| IBIS file qfp100_1p8v.ibs generated by Viper version: 2020.12.17
[IBIS Ver]   5.0
[Comment Char]   |_char
[File Name]   qfp100_1p8v.ibs
[File Rev]   1.3
[Date]   Thu Dec 17 17:51:14 2020
[Source]   NXP Viper 2020.12.17
[Notes]
[Disclaimer] IMPORTANT NOTICE
  This information is provided on an AS IS basis and without warranty.
  IN NO EVENT SHALL NXP BE LIABLE FOR INCIDENTAL OR CONSEQUENTIAL
  DAMAGES ARISING FROM USE OF THIS INFORMATION. THIS DISCLAIMER OF
  WARRANTY EXTENDS TO THE USER OF THE INFORMATION, AND TO THEIR CUSTOMERS
  OR USERS OF PRODUCTS  AND IS IN LIEU OF ALL WARRANTIES WHETHER EXPRESS,
  IMPLIED, OR STATUTORY, INCLUDING IMPLIED WARRANTIES OF MERCHANTABILITY
  OR FITNESS FOR PARTICULAR PURPOSE.
  NXP does not represent or warrant that the information furnished
  hereunder is free of infringement of any third party patents,
  copyrights, trade secrets, or other intellectual property rights.
  NXP does not represent or warrant that the information is free of
  defect, or that it meets any particular standard, requirements or need
  of the user of the infomation or their customers.
  NXP reserves the right to change the information in this file
  without notice.
   http://www.nxp.com
[Copyright]   (C) Copyright NXP 2004 - 2020, All Rights Reserved.
|   qfp100
[Component]   qfp100
[Manufacturer]   NXP
[Package]
| variable   typ   min   max
R_pkg   0.20929   0.13326   0.23511
L_pkg   4.766e-09   4.182e-09   5.347e-09
C_pkg   4.363e-13   3.854e-13   5.112e-13
[Pin] signal_name   model_name   R_pin   L_pin   C_pin
1   P2_1   gpio   0.22359   5.036e-09 4.838e-13
2   OPAMP2_INN   NC   0.21497   4.843e-09 4.817e-13
3   P1_24   gpio   0.21478   4.857e-09 4.678e-13
4   P1_7   gpio   0.218   4.970e-09 4.597e-13
5   P0_1   gpio   0.2137   4.924e-09 4.401e-13
6   P1_0   gpio   0.21171   4.894e-09 4.292e-13
7   ADC1IN1B   NC   0.20848   4.761e-09 4.267e-13
8   ADC1IN1A   NC   0.19449   4.500e-09 4.295e-13
9   P0_11   gpio   0.19424   4.487e-09 4.205e-13
10   P0_12   gpio   0.19613   4.592e-09 4.148e-13
11   P1_20   gpio   0.20355   4.669e-09 3.944e-13
12   VDDE_0   POWER   NA   NA   NA
13   VDDA   POWER   NA   NA   NA
14   VREF_OUT   NC   NA   NA   NA
15   VREFP   NC   NA   NA   NA
16   VREFN   NC   NA   NA   NA
17   VSSA   GND   NA   NA   NA
18   VSSA   GND   NA   NA   NA
19   P0_23   gpio   0.20931   4.770e-09 4.124e-13
20   P0_16   gpio   0.21094   4.801e-09 4.247e-13
21   P0_10   gpio   0.21059   4.789e-09 4.343e-13
22   P0_15   gpio   0.20486   4.653e-09 4.661e-13
23   P0_31   gpio   0.21132   4.793e-09 4.798e-13
24   P2_0   gpio   0.22019   4.963e-09 4.885e-13
25   P1_9   gpio   0.22303   5.076e-09 4.722e-13
26   P0_8   gpio   0.22345   5.084e-09 4.854e-13
27   OPAMP0_INN   NC   0.21484   4.864e-09 4.951e-13
28   P0_27   gpio   0.20723   4.771e-09 4.735e-13
29   OPAMP1_INN   NC   0.21128   4.865e-09 4.521e-13
30   P1_19   gpio   0.20854   4.878e-09 4.401e-13
31   DAC0_OUT   NC   0.206   4.816e-09 4.186e-13
32   XTAL32M_N   NC   0.20742   4.770e-09 4.123e-13
33   XTAL32M_P   NC   0.19377   4.497e-09 4.206e-13
34   RESETN   gpio   0.19458   4.551e-09 4.119e-13
35   P1_5   gpio   0.19484   4.525e-09 4.071e-13
36   P1_8   gpio   0.2033   4.733e-09 3.981e-13
37   P1_21   gpio   0.20532   4.769e-09 3.889e-13
38   VDD_CORE   POWER   NA   NA   NA
39   P1_10   gpio   0.20393   4.722e-09 3.877e-13
40   P1_22   gpio   0.20253   4.623e-09 3.978e-13
41   P0_17   gpio   0.1965   4.443e-09 4.056e-13
42   P0_7   gpio   0.19935   4.370e-09 4.202e-13
43   VDDE_2   POWER   NA   NA   NA
44   VSS_MAIN_PWR   GND   NA   NA   NA
45   VSS_MAIN   GND   NA   NA   NA
46   LX   NC   0.13326   4.182e-09 5.112e-13
47   VDD_MAIN_PWR   NC   NA   NA   NA
48   VDD_MAIN   NC   NA   NA   NA
49   P1_23   gpio   0.22732   4.889e-09 4.839e-13
50   P1_6   gpio   0.23364   5.213e-09 4.781e-13
51   XTAL32K_P   NC   0.22796   4.990e-09 4.836e-13
52   XTAL32K_N   NC   0.2234   4.815e-09 4.954e-13
53   VBAT   NC   NA   NA   NA
54   P0_0   gpio   0.22115   4.940e-09 4.485e-13
55   P0_9   gpio   0.21453   4.836e-09 4.446e-13
56   P0_18   gpio   0.21091   4.806e-09 4.328e-13
57   P1_14   gpio   0.20872   4.790e-09 4.186e-13
58   P1_13   gpio   0.19633   4.586e-09 4.144e-13
59   P1_1   gpio   0.1964   4.593e-09 4.130e-13
60   P0_26   gpio   0.19597   4.536e-09 4.137e-13
61   P1_2   gpio   0.20506   4.751e-09 4.044e-13
62   P1_3   gpio   0.2073   4.774e-09 3.901e-13
63   VDDE_4   POWER   NA   NA   NA
64   P1_18   gpio   0.20968   4.757e-09 3.946e-13
65   P1_30   gpio   0.20872   4.724e-09 4.090e-13
66   P0_28   gpio   0.20197   4.577e-09 4.097e-13
67   P1_12   gpio   0.20002   4.567e-09 4.142e-13
68   P1_26   gpio   0.20357   4.672e-09 4.224e-13
69   P0_24   gpio   0.21269   4.876e-09 4.152e-13
70   P0_13   iic   0.21536   4.889e-09 4.354e-13
71   P0_14   iic   0.2194   4.920e-09 4.378e-13
72   P1_28   gpio   0.22057   4.931e-09 4.474e-13
73   P0_20   gpio   0.2194   4.845e-09 4.688e-13
74   VDDE_4   POWER   NA   NA   NA
75   P1_4   gpio   0.23319   5.014e-09 4.840e-13
76   P0_21   gpio   0.23511   5.347e-09 4.796e-13
77   P1_25   gpio   0.22334   4.949e-09 4.943e-13
78   P0_22   gpio   0.21505   4.857e-09 4.731e-13
79   P0_25   gpio   0.22039   4.977e-09 4.534e-13
80   P1_29   gpio   0.21599   4.949e-09 4.368e-13
81   P0_2   gpio   0.21746   4.944e-09 4.295e-13
82   P1_15   gpio   0.21349   4.812e-09 4.315e-13
83   P0_19   gpio   0.19872   4.518e-09 4.316e-13
84   P0_3   gpio   0.20028   4.498e-09 4.141e-13
85   VDDE_4   POWER   NA   NA   NA
86   P1_27   gpio   0.20706   4.743e-09 3.880e-13
87   P0_4   gpio   0.2043   4.699e-09 3.854e-13
88   P1_16   gpio   0.19807   4.528e-09 4.115e-13
89   P0_6   gpio   0.20532   4.850e-09 3.921e-13
90   P0_5   gpio   0.20447   4.757e-09 3.984e-13
91   P1_17   gpio   0.19816   4.603e-09 4.099e-13
92   P1_31   gpio   0.19768   4.570e-09 4.240e-13
93   P0_29   gpio   0.20649   4.690e-09 4.278e-13
94   P1_11   gpio   0.21516   4.752e-09 4.253e-13
95   P0_30   gpio   0.21957   4.695e-09 4.329e-13
96   VDDE_4   POWER   NA   NA   NA
97   VDD3V3_USB_FS   POWER   NA   NA   NA
98   USB_FS_DP_DM_IOP   NC   0.21894   4.661e-09 4.667e-13
99   USB_FS_DP_DM_IOM   NC   0.22487   4.721e-09 4.843e-13
100   VSS_USB_FS   GND   NA   NA   NA
101   VSS   GND   NA   NA   NA
[Pin Mapping]   pulldown_ref   pullup_ref
1   VSS   VDDE_0
2   NC   NC
3   VSS   VDDE_0
4   VSS   VDDE_0
5   VSS   VDDE_0
6   VSS   VDDE_0
7   NC   NC
8   NC   NC
9   VSS   VDDE_0
10   VSS   VDDE_0
11   VSS   VDDE_0
12   NC   VDDE_0
13   NC   VDDA
14   NC   NC
15   NC   NC
16   NC   NC
17   VSSA   NC
18   VSSA   NC
19   VSS   VDDE_0
20   VSS   VDDE_0
21   VSS   VDDE_0
22   VSS   VDDE_0
23   VSS   VDDE_0
24   VSS   VDDE_0
25   VSS   VDDE_0
26   VSS   VDDE_0
27   NC   NC
28   VSS   VDDE_0
29   NC   NC
30   VSS   VDDE_0
31   NC   NC
32   NC   NC
33   NC   NC
34   VSS   VDDE_2
35   VSS   VDDE_2
36   VSS   VDDE_2
37   VSS   VDDE_2
38   NC   VDD_CORE
39   VSS   VDDE_2
40   VSS   VDDE_2
41   VSS   VDDE_2
42   VSS   VDDE_2
43   NC   VDDE_2
44   VSS_MAIN_PWR   NC
45   VSS_MAIN   NC
46   NC   NC
47   NC   NC
48   NC   NC
49   VSS   VDDE_2
50   VSS   VDDE_2
51   NC   NC
52   NC   NC
53   NC   NC
54   VSS   VDDE_4
55   VSS   VDDE_4
56   VSS   VDDE_4
57   VSS   VDDE_4
58   VSS   VDDE_4
59   VSS   VDDE_4
60   VSS   VDDE_4
61   VSS   VDDE_4
62   VSS   VDDE_4
63   NC   VDDE_4
64   VSS   VDDE_4
65   VSS   VDDE_4
66   VSS   VDDE_4
67   VSS   VDDE_4
68   VSS   VDDE_4
69   VSS   VDDE_4
70   VSS   VDDE_4
71   VSS   VDDE_4
72   VSS   VDDE_4
73   VSS   VDDE_4
74   NC   VDDE_4
75   VSS   VDDE_4
76   VSS   VDDE_4
77   VSS   VDDE_4
78   VSS   VDDE_4
79   VSS   VDDE_4
80   VSS   VDDE_4
81   VSS   VDDE_4
82   VSS   VDDE_4
83   VSS   VDDE_4
84   VSS   VDDE_4
85   NC   VDDE_4
86   VSS   VDDE_4
87   VSS   VDDE_4
88   VSS   VDDE_4
89   VSS   VDDE_4
90   VSS   VDDE_4
91   VSS   VDDE_4
92   VSS   VDDE_4
93   VSS   VDDE_4
94   VSS   VDDE_4
95   VSS   VDDE_4
96   NC   VDDE_4
97   NC   VDD3V3_USB_FS
98   NC   NC
99   NC   NC
100   VSS_USB_FS   NC
101   VSS   NC
|*   Model Selector   *
[Model Selector] gpio
MFIO1V8_pd_hs   EPUN=1 EPD=1 EHS=1
MFIO1V8_pd_ls   EPUN=1 EPD=1 EHS=0
MFIO1V8_pu_hs   EPUN=0 EPD=0 EHS=1
MFIO1V8_pu_ls   EPUN=0 EPD=0 EHS=0
MFIO1V8_p_hs   EPUN=1 EPD=0 EHS=1
MFIO1V8_p_ls   EPUN=1 EPD=0 EHS=0
MFIO1V8_r_hs   EPUN=0 EPD=1 EHS=1
MFIO1V8_r_ls   EPUN=0 EPD=1 EHS=0
[Model Selector] iic
IIC1V8_pd_hs   EGP=1 EPUN=1 EPD=1 EHS=1
IIC1V8_pd_ls   EGP=1 EPUN=1 EPD=1 EHS=0
IIC1V8_p_hs   EGP=1 EPUN=1 EPD=0 EHS=1
IIC1V8_p_ls   EGP=1 EPUN=1 EPD=0 EHS=0
IIC1V8_pu_hs   EGP=1 EPUN=0 EPD=0 EHS=1
IIC1V8_pu_ls   EGP=1 EPUN=0 EPD=0 EHS=0
IIC1V8_r_hs   EGP=1 EPUN=0 EPD=1 EHS=1
IIC1V8_r_ls   EGP=1 EPUN=0 EPD=1 EHS=0
IIC1V8_pd_iic_hs   EGP=0 ECS=0 EPUN=1 EPD=1
IIC1V8_p_iic_hs   EGP=0 ECS=0 EPUN=1 EPD=0
IIC1V8_pu_iic_hs   EGP=0 ECS=0 EPUN=0 EPD=0
IIC1V8_r_iic_hs   EGP=0 ECS=0 EPUN=0 EPD=1
IIC1V8_pd_iic_pu_hs   EGP=0 ECS=1 EPUN=1 EPD=1 SSEL=1
IIC1V8_p_iic_pu_hs   EGP=0 ECS=1 EPUN=1 EPD=0 SSEL=1
IIC1V8_pu_iic_pu_hs   EGP=0 ECS=1 EPUN=0 EPD=0 SSEL=1
IIC1V8_r_iic_pu_hs   EGP=0 ECS=1 EPUN=0 EPD=1 SSEL=1
| End [Component] qfp100
| Models and submodels in the file (24): IIC1V8_p_hs (I/O), IIC1V8_p_iic_hs (I/O_open_drain), IIC1V8_p_iic_pu_hs (I/O_open_drain), IIC1V8_p_ls (I/O), IIC1V8_pd_hs (I/O), IIC1V8_pd_iic_hs (I/O_open_drain), IIC1V8_pd_iic_pu_hs (I/O_open_drain), IIC1V8_pd_ls (I/O), IIC1V8_pu_hs (I/O), IIC1V8_pu_iic_hs (I/O_open_drain), IIC1V8_pu_iic_pu_hs (I/O_open_drain), IIC1V8_pu_ls (I/O), IIC1V8_r_hs (I/O), IIC1V8_r_iic_hs (I/O_open_drain), IIC1V8_r_iic_pu_hs (I/O_open_drain), IIC1V8_r_ls (I/O), MFIO1V8_p_hs (I/O), MFIO1V8_p_ls (I/O), MFIO1V8_pd_hs (I/O), MFIO1V8_pd_ls (I/O), MFIO1V8_pu_hs (I/O), MFIO1V8_pu_ls (I/O), MFIO1V8_r_hs (I/O), MFIO1V8_r_ls (I/O)
